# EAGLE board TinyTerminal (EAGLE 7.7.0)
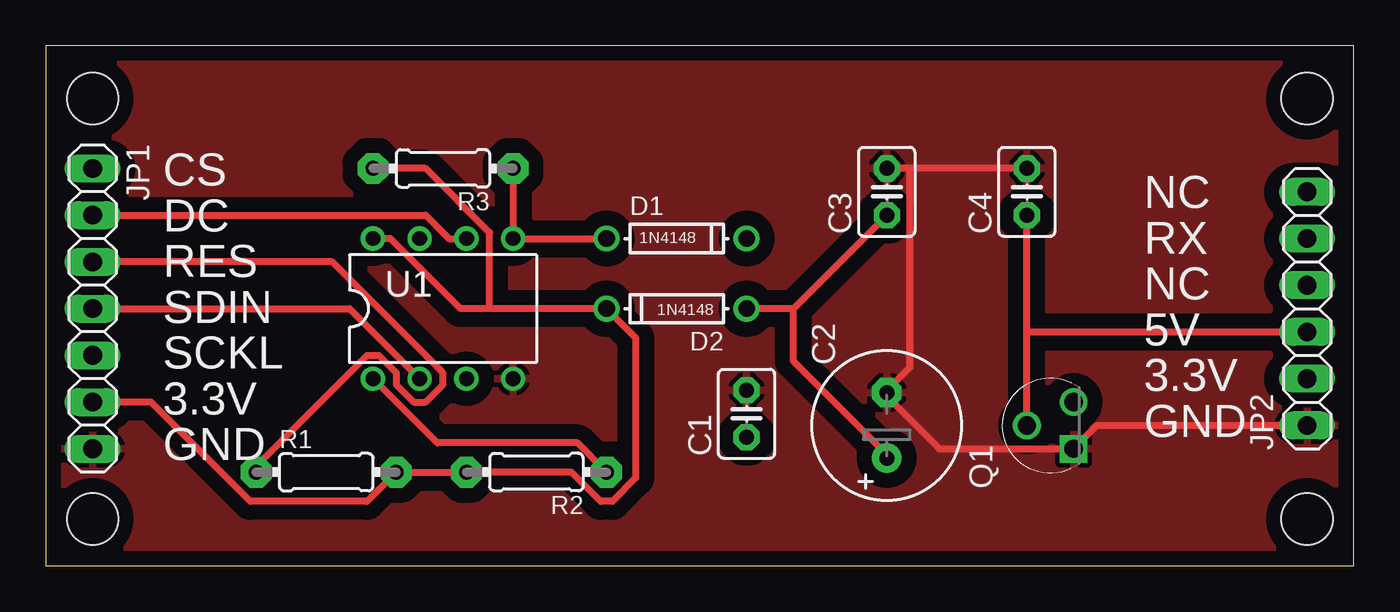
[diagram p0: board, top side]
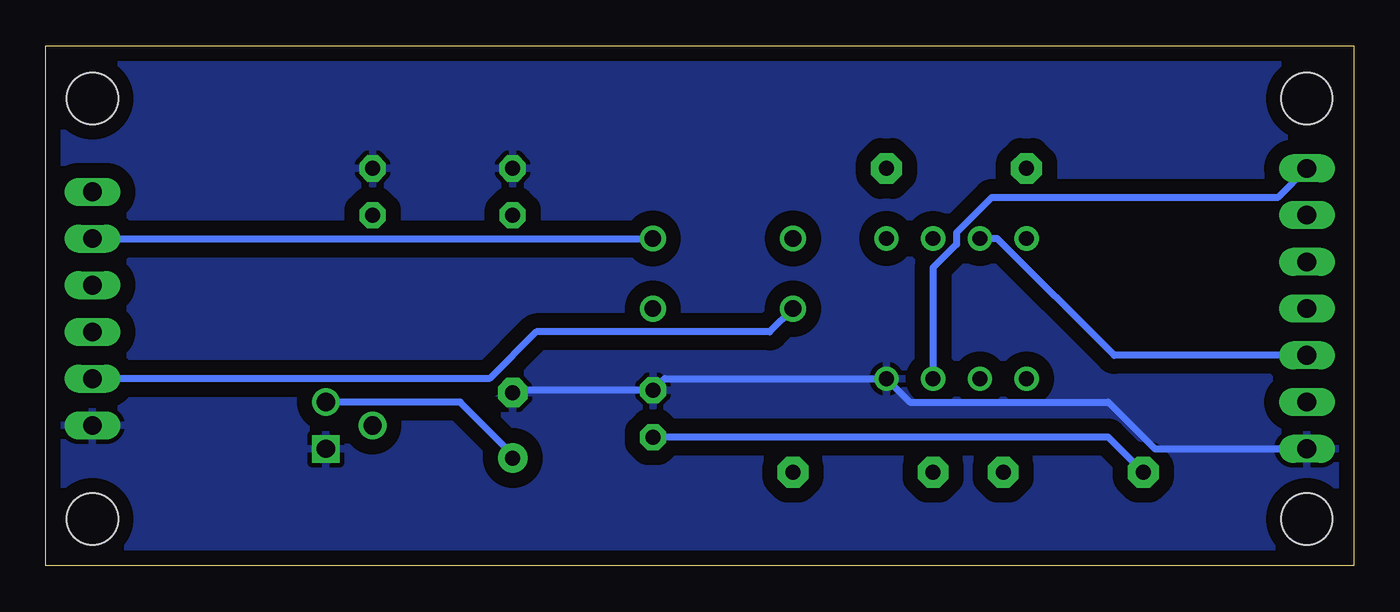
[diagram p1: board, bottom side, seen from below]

Size 71.1 x 28.24 mm. Coordinates in mm from the lower left corner, seen from the top.
Outline: 0,0 71.1,0 71.1,28.24 0,28.24 0,0
Copper layers (1*16): Top 0.035mm / dielectric 1.5mm / Bottom 0.035mm
Design rules "ITEADstudio_GB_DRC": minimum track width 10mil, minimum drill 12mil, track to track 10mil, track to pad 10mil, pad to pad 6mil, via to via 10mil, smd to smd 0mil, copper to edge 10mil, drill to drill 10mil, minimum pad ring 10mil, minimum via ring 6mil, stop-mask expansion 2mil, vias tented up to drill 100mil, thermal gap 10mil
Net classes: 0 GND: width 0.381 mm; 1 VCC: width 0.381 mm; 2 5V: width 0.381 mm
Holes 2.8 mm at 2.54,25.4 2.54,2.54 68.58,2.54 68.58,25.4

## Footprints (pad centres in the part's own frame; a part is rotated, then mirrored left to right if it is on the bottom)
C025-030X050 = drill 0.813 pad 1.422 octagon: 1 -1.27,0; 2 1.27,0
E3,5-8 = drill 0.813 pad 1.6: + -1.778,0 | drill 0.813 pad 1.6 octagon: - 1.778,0
DO-1N4148 = drill 0.9: A -3.81,0; C 3.81,0
1X07 = drill 1.016 long: 1 -7.62,0; 2 -5.08,0; 3 -2.54,0; 4 0,0; 5 2.54,0; 6 5.08,0; 7 7.62,0
1X06 = drill 1.016 long: 1 -6.35,0; 2 -3.81,0; 3 -1.27,0; 4 1.27,0; 5 3.81,0; 6 6.35,0
TO127P254X533-3 = drill 0.991 square: 1 -2.54,-2.54 | drill 0.991: 2 -1.27,0; 3 0,-2.54
0204/7 = drill 0.813 pad 1.676 octagon: 1 -3.81,0; 2 3.81,0
PDIP08_300MIL = drill 0.813: 1 -3.81,-3.81; 2 -1.27,-3.81; 3 1.27,-3.81; 4 3.81,-3.81; 5 3.81,3.81; 6 1.27,3.81; 7 -1.27,3.81; 8 -3.81,3.81

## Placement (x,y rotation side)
C1  100nF  [C025-030X050]  38.1,8.25 90 top
C2  2.2μF  [E3,5-8]  45.72,7.62 90 top
C3  100 nF  [C025-030X050]  45.72,20.32 90 top
C4  100 nF  [C025-030X050]  53.34,20.32 90 top
D1  1N4148  [DO-1N4148]  34.29,17.78 0 top
D2  1N4148  [DO-1N4148]  34.29,13.97 180 top
JP1  [1X07]  2.54,13.97 270 top
JP2  [1X06]  68.58,13.97 90 top
Q1  MCP1702-3302E/TO  [TO127P254X533-3]  53.34,8.89 90 top
R1  33K  [0204/7]  15.24,5.08 0 top
R2  10K  [0204/7]  26.67,5.08 180 top
R3  10K  [0204/7]  21.59,21.59 180 top
U1  ATTINY85-P  [PDIP08_300MIL]  21.59,13.97 0 top

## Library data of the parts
C1-C4 D1 D2 R1-R3 = adafruit
JP1 JP2 = pinhead
Q1 = MCP1702-3302E_TO; AVAILABILITY: Unavailable; DESCRIPTION: Low Iq 250mA LDO, Vin 13.2V max, Vout=3.3V 3 TO-92 2x3mm BAG ; RoHS Compliant: Yes; MF: Microchip; MP: MCP1702-3302E/TO; PACKAGE: TO-92 Microchip; PRICE: None
U1 = atmel_attiny25_45_85

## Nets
5V: C4.1 JP2.3 Q1.2
GND: C1.2 C2.- C3.2 C4.2 JP1.7 JP2.1 Q1.1 U1.4
N$1: JP1.5 U1.7
N$2: JP1.4 U1.2
N$3: JP1.2 U1.6
N$4: JP1.1 U1.3
N$5: D1.C JP2.5
N$6: D1.A R3.1 U1.5
N$7: C2.+ C3.1 D2.A Q1.3
N$8: C1.1 JP1.3 R1.1
N$9: R2.1 U1.1
VCC: D2.C JP1.6 JP2.2 R1.2 R2.2 R3.2 U1.8

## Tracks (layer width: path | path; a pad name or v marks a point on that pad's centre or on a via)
5V
  Top 0.381: Q1.2 53.34,12.7 | 53.34,12.7 C4.1 | 53.34,12.7 JP2.3
GND
  Top 0.381: C4.2 46.99,21.59 | 46.99,21.59 C3.2 | JP2.1 57.15,7.62 Q1.1 48.58,6.35 45.72,9.21 C2.- 45.72,9.53 46.99,10.8 46.99,21.59
  Bottom 0.381: JP1.7 10.79,6.35 13.34,8.89 24.13,8.89 U1.4 37.47,10.16 C1.2 45.72,9.53 C2.-
  pour Bottom (isolate 0.813): 0,27.94 71.12,27.94 71.12,0 0,0
  pour Top (isolate 0.813): 0,27.94 71.12,27.94 71.12,0 0,0
N$1
  Bottom 0.381: U1.7 19.37,17.78 13.02,11.43 JP1.5
N$2
  Top 0.381: U1.2 16.51,13.97 JP1.4
N$3
  Top 0.381: U1.6 21.91,17.78 20.64,19.05 JP1.2
N$4
  Bottom 0.381: U1.3 22.86,16.19 21.59,17.46 21.59,18.1 19.68,20 4.13,20 JP1.1
N$5
  Bottom 0.381: JP2.5 D1.C
N$6
  Top 0.381: R3.1 U1.5 D1.A
N$7
  Top 0.381: 40.64,13.97 D2.A | C3.1 40.64,13.97 | 40.64,13.97 40.64,11.11 45.72,6.03 C2.+
  Bottom 0.381: Q1.3 48.58,8.89 45.72,6.03 C2.+
N$8
  Top 0.381: JP1.3 15.56,16.51 21.59,10.48 21.59,9.84 20.64,8.89 20,8.89 19.05,9.84 19.05,10.48 18.1,11.43 17.46,11.43 11.43,5.4 R1.1
  Bottom 0.381: C1.1 13.34,6.99 R1.1
N$9
  Top 0.381: U1.1 21.27,6.67 28.89,6.67 R2.1
VCC
  Top 0.381: JP1.6 5.71,8.89 11.11,3.49 17.46,3.49 R1.2 R2.2 28.57,5.08 30.16,3.49 30.8,3.49 32.07,4.76 32.07,12.38 D2.C 24.13,13.97 | U1.8 18.73,17.78 22.54,13.97 24.13,13.97 | R3.2 20.64,21.59 24.13,18.1 24.13,13.97
  Bottom 0.381: JP2.2 46.99,10.16 44.45,12.7 31.75,12.7 D2.C

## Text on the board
tNames: NC / RX / NC / 5V / 3.3V / GND | CS / DC / RES / SDIN / SCKL / 3.3V / GND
